TYPE "stSCTMi_Ejector"
VERSION : 0.1
  STRUCT
   btErrorByte : BYTE ;
   btWarningByte : BYTE ;
   btLeakageOfLastCycle : BYTE ;
   wSystemVacuum : WORD ;
   wEvacuationTimeT1 : WORD ;
   wLastFreeFlowVacuum : WORD ;
   wAirConsumptionOfLastCyc : WORD ;
   bAirSavingFunktion_H1 : BOOL ;
   bPartPresent_H2 : BOOL ;
  END_STRUCT ;
END_TYPE

